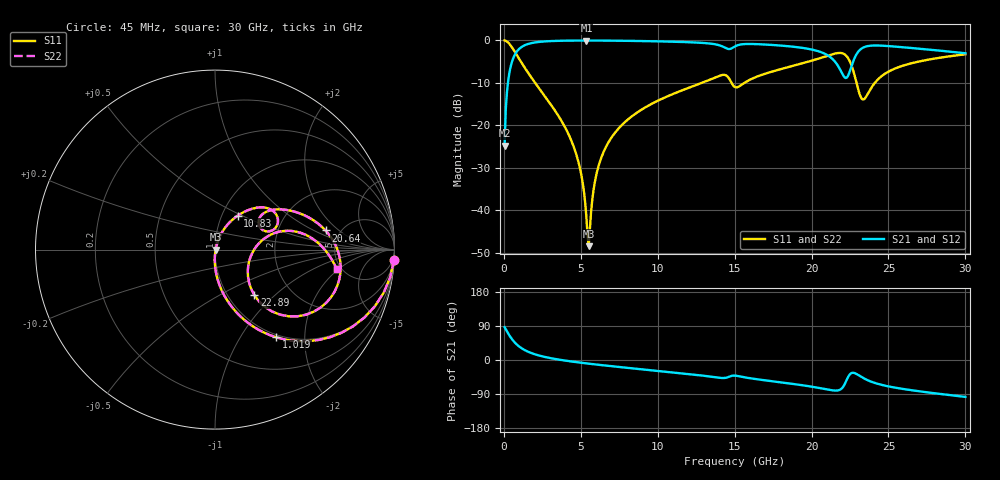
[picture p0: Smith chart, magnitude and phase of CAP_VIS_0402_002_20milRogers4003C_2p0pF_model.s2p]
! S-parameter model data by Modelithics Inc.  support@modelithics.com  813-866-6335  Tampa FL USA
! S-Parameter data specifications:
! Substrate: 20-mil Rogers 4003C, substrate thickness, H=0.508mm, Dielectric constant, Er=3.75
! PCB Mounting Pad Footprint: Pad width, PadW=0.50mm , Pad length, PadL=0.50mm , Pad gap, PadG (edge-to-edge)=0.40mm , Reference planes=1.4mm apart
! Created Wed Nov 18 12:44:05 2015
# hz S ma R 50
! 2 Port Network Data from SP1.SP block
! freq  magS11  angS11  magS21  angS21  magS12  angS12  magS22  angS22
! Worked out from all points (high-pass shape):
!   401 points, 45 MHz to 30 GHz, reference 50 ohm
!   highest |S21| = -0.03 dB at 5.362 GHz (marker M1); lowest = -24.8 dB at 45 MHz (marker M2)
!   |S21| within 3 dB of the highest: 765.9 MHz to 20.79 GHz (20.03 GHz wide, 186 % of centre); 22.96 GHz to end of sweep
!   lowest |S11| = -48.5 dB at 5.512 GHz (marker M3), VSWR 1.01, Z = 50.4 - j0.00158 ohm
!   |S11| at or under -10 dB: 2.029 GHz to 12.87 GHz (10.84 GHz wide, 146 % of centre); 14.8 GHz to 15.64 GHz (838.4 MHz wide, 5.51 % of centre); 22.92 GHz to 24.12 GHz (1.192 GHz wide, 5.07 % of centre)
!   |S22| runs from -48.5 to 0.0 dB; largest |S21 - S12| = 0
!   S11 on the Smith chart (normalised r, x): 45 MHz: 1, -34; 1.019 GHz: 0.96, -1.45; 10.83 GHz: 1.19, +0.47; 20.64 GHz: 3.83, +1.34; 22.89 GHz: 1.32, -0.76; 30 GHz: 4.57, -1.88
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4.5e7  0.9983 -3.4  0.05747 86.6  0.05747 86.6  0.9983 -3.4
4.194375e8  0.8799 -29.1  0.4747 60.9  0.4747 60.9  0.8799 -29.1
1.018538e9  0.5952 -55.1  0.8022 34.7  0.8022 34.7  0.5952 -55.1
2.066962e9  0.3094 -75.2  0.9487 14.4  0.9487 14.4  0.3094 -75.2
4.014038e9  0.09175 -89.8  0.9926 -1.8  0.9926 -1.8  0.09175 -89.8
5.062462e9  0.02432 -89.1  0.996 -7.5  0.996 -7.5  0.02432 -89.1
5.362012e9  0.00825 -72.6  0.9961 -9.0  0.9961 -9.0  0.00825 -72.6
5.511788e9  0.003768 -0.2  0.9961 -9.7  0.9961 -9.7  0.003768 -0.2
6.036e9  0.02753 69.7  0.9955 -12.1  0.9955 -12.1  0.02753 69.7
6.709988e9  0.05911 70.8  0.9939 -15.1  0.9939 -15.1  0.05911 70.8
1.007992e10  0.1976 59.3  0.9741 -29.0  0.9741 -29.0  0.1976 59.3
1.08288e10  0.2273 56.3  0.9669 -32.1  0.9669 -32.1  0.2273 56.3
1.419874e10  0.3916 31.8  0.8495 -47.5  0.8495 -47.5  0.3916 31.8
1.50225e10  0.2818 24.6  0.8504 -41.2  0.8504 -41.2  0.2818 24.6
2.003996e10  0.5792 15.8  0.7786 -70.6  0.7786 -70.6  0.5792 15.8
2.063906e10  0.625 9.8  0.7242 -74.9  0.7242 -74.9  0.625 9.8
2.191215e10  0.7104 -16.5  0.4338 -76.8  0.4338 -76.8  0.7104 -16.5
2.243636e10  0.5908 -39.0  0.4086 -40.6  0.4086 -40.6  0.5908 -39.0
2.288569e10  0.3365 -49.2  0.6685 -36.1  0.6685 -36.1  0.3365 -49.2
2.34099e10  0.2026 -10.8  0.8314 -48.6  0.8314 -48.6  0.2026 -10.8
2.505742e10  0.4342 13.9  0.8558 -70.1  0.8558 -70.1  0.4342 13.9
3e10  0.6864 -9.1  0.7053 -97.4  0.7053 -97.4  0.6864 -9.1
